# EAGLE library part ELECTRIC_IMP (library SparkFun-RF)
Electric Imp SD Socket The Electric Imp provides an easy, integrated way to connect almost any hardware device both to other devices and to internet services. It’s more than just a WiFi card, or even a WiFi module with processing built in - it’s an integrated platform that deals with the drudgery of connectivity, allowing you to concentrate on the application instead of the mechanics. This device matches the Electric Imp pinout to a 4UCONN SD MMC connector. The 4UCONN part number for the connector is 19646. SparkFun Products: Electric Imp Breakout (WRL-12886) SparkFun Electric Imp Shield (WRL-12887)
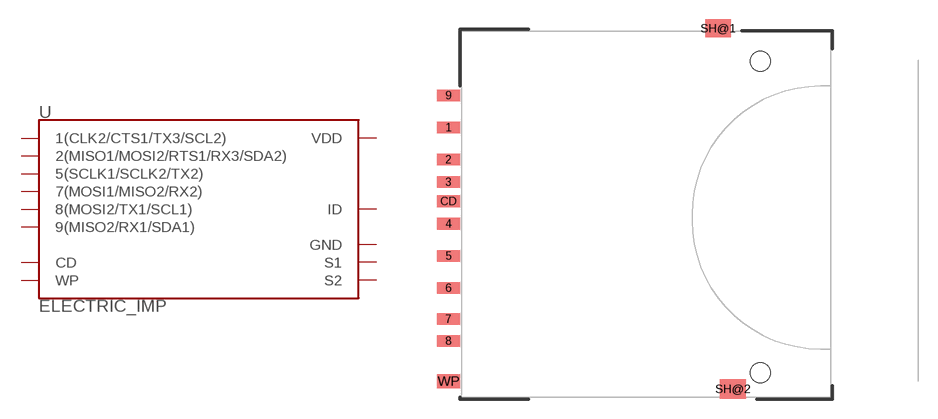
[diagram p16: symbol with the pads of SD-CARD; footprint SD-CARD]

Designator prefix U

## ELECTRIC_IMP (PROD_ID: CONN-11976)  [SD-CARD]
1  1(CLK2/CTS1/TX3/SCL2)
2  2(MISO1/MOSI2/RTS1/RX3/SDA2)
3  GND
4  VDD
5  5(SCLK1/SCLK2/TX2)
6  ID
7  7(MOSI1/MISO2/RX2)
8  8(MOSI2/TX1/SCL1)
9  9(MISO2/RX1/SDA1)
CD  CD
SH@1  S1
SH@2  S2
WP  WP

## Footprint SD-CARD (pad centres in mm)
SD Card Socket The 4UCONN part number is 19646. See this part in action on the Electric Imp Breakout.
smd 1.8 x 0.9: 1 -1,6.77; 2 -1,4.27; 3 -1,2.52; 4 -1,-0.73; 5 -1,-3.23; 6 -1,-5.73; 7 -1,-8.15; 8 -1,-9.85; 9 -1,9.27; CD -1,1.02
smd 2 x 1.4: SH@1 20,14.496
smd 2 x 1.527: SH@2 21.15,-13.589
smd 1.8 x 1.1: WP -1,-13
hole 1.55 at 23.3,11.94
hole 1.55 at 23.3,-12.32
